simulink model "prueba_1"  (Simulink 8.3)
settings: Solver=ode45  StartTime=0.0  StopTime=inf  RelTol=1e-3
PreLoadFcn:
  | m=10
  | l=5
  | g=9.81
  | b=2
undefined symbols (not defined in the file or in its folder): magnitude
libraries: simulink x1

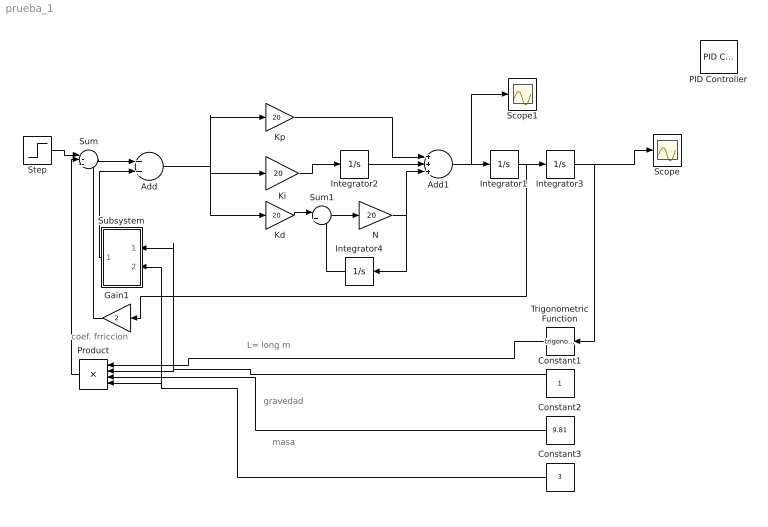
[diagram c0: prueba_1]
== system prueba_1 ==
  note: masa
  note: gravedad
  note: coef. frriccion
  note: L= long m
  Add : Sum
  Add1 : Sum  Inputs=+++
  Constant1 : Constant
  Constant2 : Constant  Value=9.81
  Constant3 : Constant  Value=3
  Gain1 : Gain  Gain=2
  Integrator1 : Integrator  InitialCondition=1
  Integrator2 : Integrator
  Integrator3 : Integrator
  Integrator4 : Integrator
  Kd : Gain  Gain=20
  Ki : Gain  Gain=20
  Kp : Gain  Gain=20
  N : Gain  Gain=20
  PID Controller : simulink/Continuous/PID Controller  Controller=P  TimeDomain=Continuous-time  SampleTime=1  IntegratorMethod=Forward Euler  FilterMethod=Forward Euler  Form=Parallel  P=5  I=11  D=0  N=100  InitialConditionSource=internal  InitialConditionForIntegrator=0  InitialConditionForFilter=0  ExternalReset=none  LimitOutput=off  UpperSaturationLimit=inf  LowerSaturationLimit=-inf  LinearizeAsGain=on  AntiWindupMode=none  Kb=1  TrackingMode=off  Kt=1  PParamMin=[]  PParamMax=[]  IParamMin=[]  IParamMax=[]  DParamMin=[]  DParamMax=[]  NParamMin=[]  NParamMax=[]  KbParamMin=[]  KbParamMax=[]  KtParamMin=[]  KtParamMax=[]  POutMin=[]  POutMax=[]  IOutMin=[]  IOutMax=[]  DOutMin=[]  DOutMax=[]  NOutMin=[]  NOutMax=[]  KbOutMin=[]  KbOutMax=[]  KtOutMin=[]  KtOutMax=[]  IntegratorOutMin=[]  IntegratorOutMax=[]  FilterOutMin=[]  FilterOutMax=[]  SumOutMin=[]  SumOutMax=[]  SumI1OutMin=[]  SumI1OutMax=[]  SumI2OutMin=[]  SumI2OutMax=[]  SumI3OutMin=[]  SumI3OutMax=[]  SumDOutMin=[]  SumDOutMax=[]  SaturationOutMin=[]  SaturationOutMax=[]  IntegratorContinuousStateAttributes=''  IntegratorStateMustResolveToSignalObject=off  IntegratorRTWStateStorageClass=Auto  FilterContinuousStateAttributes=''  FilterStateMustResolveToSignalObject=off  FilterRTWStateStorageClass=Auto
  Product : Product  Inputs=4
  Scope : Scope
  Scope1 : Scope
  Step : Step  Time=0  SampleTime=0
  Subsystem : Subsystem
  Sum : Sum  Inputs=|+--
  Sum1 : Sum  Inputs=|+-
  Trigonometric Function : Trigonometry
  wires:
  Step/1 -> Sum/1
  Gain1/1 -> Sum/3
  Constant1/1 -> Product/2, Subsystem/1(In1)
  Constant2/1 -> Product/3
  Constant3/1 -> Subsystem/2(In2), Product/4
  Product/1 -> Sum/2
  Trigonometric Function/1 -> Product/1
  Sum/1 -> Add/1
  Subsystem/1(Out1) -> Add/2
  Integrator1/1 -> Gain1/1, Integrator3/1
  Integrator3/1 -> Scope/1, Trigonometric Function/1
  Ki/1 -> Integrator2/1
  Integrator2/1 -> Add1/2
  Kd/1 -> Sum1/1
  Sum1/1 -> N/1
  N/1 -> Add1/3, Integrator4/1
  Integrator4/1 -> Sum1/2
  Add/1 -> Kd/1, Ki/1, Kp/1
  Add1/1 -> Scope1/1, Integrator1/1
  Kp/1 -> Add1/1

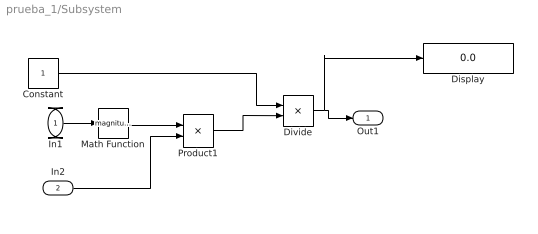
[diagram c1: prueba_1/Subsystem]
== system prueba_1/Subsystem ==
  In1 : Inport
  In2 : Inport  Port=2
  Constant : Constant
  Display : Display
  Divide : Product  Inputs=*/
  Math Function : Math  Operator=magnitude^2
  Product1 : Product
  Out1 : Outport
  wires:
  Constant/1 -> Divide/1
  Divide/1 -> Display/1, Out1/1
  In1/1 -> Math Function/1
  Math Function/1 -> Product1/1
  In2/1 -> Product1/2
  Product1/1 -> Divide/2
